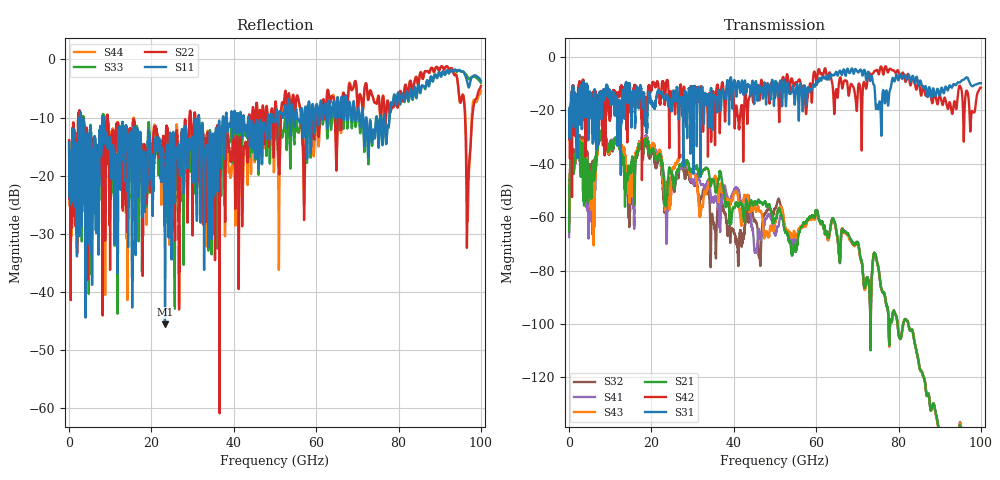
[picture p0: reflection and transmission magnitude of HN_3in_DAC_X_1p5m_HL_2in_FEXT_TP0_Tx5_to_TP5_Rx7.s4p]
# GHz S RI R 45
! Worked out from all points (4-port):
!   4000 points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, 25 MHz to 100 GHz, reference 45 ohm
!   strongest paths, dB at 25 MHz, 25.02 GHz, 50.02 GHz, 75.03 GHz, 100 GHz:
!     S31: -20.8, -20.1, -10.1, -19.6, -9.9
!     S42: -20.8, -16.2, -15.1, -5.7, -11.5
!     S21: -65.4, -43.8, -60.6, -78.3, -191.8
!     S43: -62.4, -42.6, -62.3, -78.2, -199.8
!     S41: -67.5, -44.7, -66.2, -78.2, -197.6
!     S32: -62.3, -47.4, -56.7, -78.3, -193.9
!   lowest |S11| = -45.6 dB at 23.3 GHz (marker M1), VSWR 1.01, Z = 44.8 - j0.441 ohm
!   |S11| at or under -10 dB: 2.878 GHz to 8.172 GHz (5.294 GHz wide, 95.8 % of centre); 8.307 GHz to 31.39 GHz (23.09 GHz wide, 116 % of centre); 31.58 GHz to 37.34 GHz (5.765 GHz wide, 16.7 % of centre)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
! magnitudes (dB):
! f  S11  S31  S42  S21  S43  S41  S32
! 25 MHz  -14.2  -20.8  -20.8  -65.4  -62.4  -67.5  -62.3
! 2.025 GHz  -20.9  -28.8  -18.1  -32.7  -30.9  -33.0  -30.4
! 8.3 GHz  -9.8  -13.3  -19.1  -29.8  -30.6  -30.3  -29.8
! 23.3 GHz  -45.6  -14.7  -17.8  -54.3  -57.4  -49.5  -54.9
! 91.72 GHz  -1.9  -11.9  -18.2  -155.6  -156.6  -156.5  -155.7
! 96.88 GHz  -4.5  -8.1  -14.0  -163.2  -186.9  -186.3  -164.0
! 100 GHz  -3.6  -9.9  -11.5  -191.8  -199.8  -197.6  -193.9
